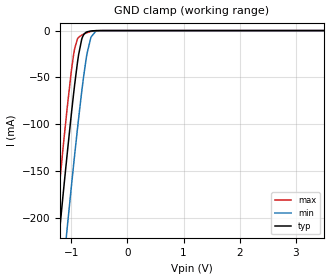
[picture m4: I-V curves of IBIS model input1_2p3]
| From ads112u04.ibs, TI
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|   input1_2p3 Model
[Model]   input1_2p3
Model_type   Input
Vinl = 0.69
Vinh = 1.61
|   typ   min   max
C_comp   6.78646E-13   6.36283E-13   7.17205E-13
[Model spec]
|subparameter
Vinl   0.69   0.6897   0.6903
Vinh   1.61   1.6093   1.6107
| Where Nom  PVT is Nominal Process, 2.3V, 27C
|   Fast PVT is Strong Process,  2.301V, -40C
|   Slow PVT is Weak Process,   2.299, 125C
[Voltage Range]   2.3   2.299   2.301
[Temperature Range]   27   125   -40
[Power Clamp Reference]   2.3   2.299   2.301
[GND Clamp Reference]   0   0   0
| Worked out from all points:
|   GND clamp passes 1 mA (typ) near -0.70 V on its own axis
[GND Clamp]
|   Voltage   I(typ)   I(min)   I(max)
-2.3V     -914.9mA   -992.5mA   -866.7mA
-1.382V   -321.3mA   -401.4mA   -270.9mA
-1.155V   -179.7mA   -259.6mA   -129.5mA
-1.072V   -130.2mA   -209.4mA   -81.15mA
-995.9mV  -86.8mA    -164.3mA   -41.23mA
-940.7mV  -57.44mA   -132.5mA   -19.04mA
-871.7mV  -26.08mA   -94.28mA   -7.305mA
-816.5mV  -9.537mA   -65.77mA   -4.877mA
-740.6mV  -1.91mA    -31.86mA   -2.726mA
-650.9mV  -406.8uA   -7.043mA   -910.5uA
-519.8mV  -22.13uA   -233uA     -44.58uA
4.6V      0A         0A         0A
[POWER Clamp]
|   Voltage   I(typ)   I(min)   I(max)
-2.3V     0A         0A         0A
0V        0A         0A         0A
4.6V      0A         0A         0A
